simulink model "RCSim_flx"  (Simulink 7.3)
settings: Solver=ode45  StartTime=0.0  StopTime=12  RelTol=1e-3
InitFcn:
  | [Av,Bv,Cv,Dv]= vehi_roll_flx;
StopFcn:
  | pl
undefined symbols (not defined in the file or in its folder): Av, Bv, Cv, Dv, Jet_Con

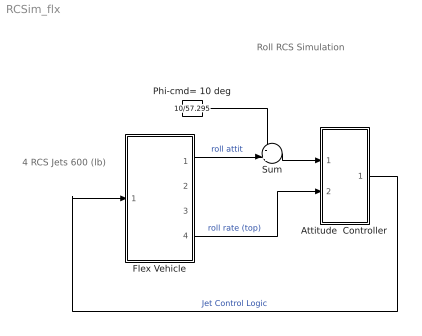
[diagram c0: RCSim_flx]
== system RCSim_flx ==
  note: Roll RCS Simulation
  note: 4 RCS Jets 600 (lb)
  Attitude  Controller : Subsystem
  Flex Vehicle : Subsystem
  Phi-cmd= 10 deg : Constant  Value=10/57.295  OutDataType=sfix(16)  OutScaling=2^0
  Sum : Sum  Inputs=-+|  OutDataType=sfix(16)  OutScaling=2^0
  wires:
  Sum/1 -> Attitude  Controller/1(ater)
  Phi-cmd= 10 deg/1 -> Sum/1
  Attitude  Controller/1(Thro) -> Flex Vehicle/1(Thr)  "Jet Control Logic"
  Flex Vehicle/4(p-flx2) -> Attitude  Controller/2(p)  "roll rate (top)"
  Flex Vehicle/1(phi) -> Sum/2  "roll attit"

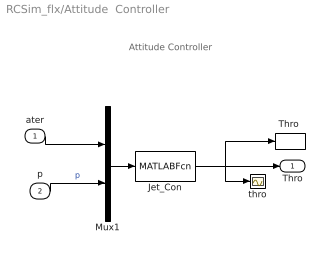
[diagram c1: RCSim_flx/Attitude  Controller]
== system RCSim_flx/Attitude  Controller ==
  note: Attitude Controller
  ater : Inport  OutDataType=sfix(16)  OutScaling=2^0
  p : Inport  Port=2  OutDataType=sfix(16)  OutScaling=2^0
  Jet_Con : MATLABFcn  MATLABFcn=Jet_Con( u(1), u(2) )  OutputDimensions=4
  Mux1 : Mux  Inputs=[1,1]
  "Thro " : ToWorkspace  VariableName=Thro  SampleTime=-1  SaveFormat=Array
  thro : Scope
  Thro : Outport  OutDataType=sfix(16)  OutScaling=2^0
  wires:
  Mux1/1 -> Jet_Con/1
  p/1 -> Mux1/2  "p"
  ater/1 -> Mux1/1
  Jet_Con/1 -> Thro/1, "Thro "/1, thro/1

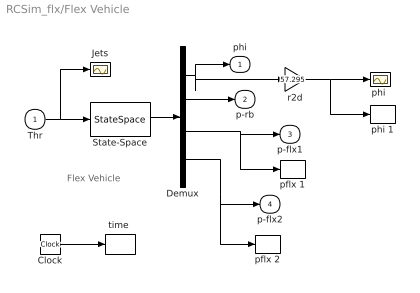
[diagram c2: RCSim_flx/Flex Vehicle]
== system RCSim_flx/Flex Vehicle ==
  note: Flex Vehicle
  Thr : Inport  PortDimensions=4  OutDataType=sfix(16)  OutScaling=2^0
  Clock : Clock
  Demux : Demux
  Jets : Scope
  State-Space : StateSpace  A=Av  B=Bv  C=Cv  D=Dv
  pflx 1 : ToWorkspace  VariableName=p1  SampleTime=-1  SaveFormat=Array
  pflx 2 : ToWorkspace  VariableName=p2  SampleTime=-1  SaveFormat=Array
  "phi " : Scope
  phi 1 : ToWorkspace  VariableName=phi  SampleTime=-1  SaveFormat=Array
  r2d : Gain  Gain=57.295  ParameterDataType=sfix(16)  ParameterScaling=2^0  OutDataType=sfix(16)  OutScaling=2^0
  "time " : ToWorkspace  VariableName=time  SampleTime=-1  SaveFormat=Array
  phi : Outport  OutDataType=sfix(16)  OutScaling=2^0
  p-rb : Outport  Port=2  OutDataType=sfix(16)  OutScaling=2^0
  p-flx1 : Outport  Port=3  OutDataType=sfix(16)  OutScaling=2^0
  p-flx2 : Outport  Port=4  OutDataType=sfix(16)  OutScaling=2^0
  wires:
  State-Space/1 -> Demux/1
  Demux/1 -> phi/1, r2d/1
  Demux/2 -> p-rb/1
  Demux/3 -> p-flx1/1, pflx 1/1
  Demux/4 -> p-flx2/1, pflx 2/1
  Thr/1 -> State-Space/1, Jets/1
  Clock/1 -> "time "/1
  r2d/1 -> "phi "/1, phi 1/1
